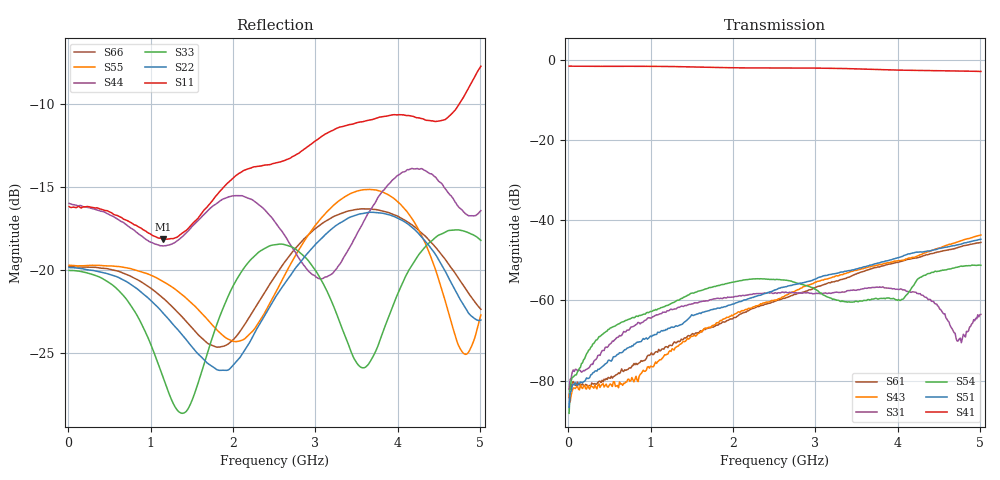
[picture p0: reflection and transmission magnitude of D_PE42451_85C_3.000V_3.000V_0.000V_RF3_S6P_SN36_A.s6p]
! Device ID: PE42451
! Serial: 36
! Insertion: A
! Temp: 85C
! VDD: 3.000
! Control_Hi: 100.000
! Control_Lo: 0.000
! Logic State: RF3
! Port 1: RFC
! Port 2: RF1
! Port 3: RF2
! Port 4: RF3
! Port 5: RF4
! Port 6: RF5
! V1 = 3.00
! V2 = 3.00
! V3 = 0.00
! V4 = 0.00
! IDD: 1.398150e-05
#  Hz  S  RI  R  50
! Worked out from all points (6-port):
!   401 points, 10 MHz to 5.01 GHz, reference 50 ohm
!   strongest paths, dB at 10 MHz, 1.26 GHz, 2.51 GHz, 3.76 GHz, 5.01 GHz:
!     S41: -1.6, -1.7, -2.1, -2.4, -2.9
!     S51: -86.6, -66.6, -57.4, -50.7, -44.8
!     S54: -88.2, -60.7, -54.9, -59.7, -51.3
!     S31: -82.1, -62.3, -58.1, -56.7, -63.5
!     S43: -83.6, -72.1, -59.9, -51.2, -43.7
!     S61: -84.0, -71.3, -60.2, -51.6, -45.6
!   lowest |S11| = -18.1 dB at 1.147 GHz (marker M1), VSWR 1.28, Z = 57.7 - j11 ohm
!   |S11| at or under -10 dB: start of sweep to 4.744 GHz
